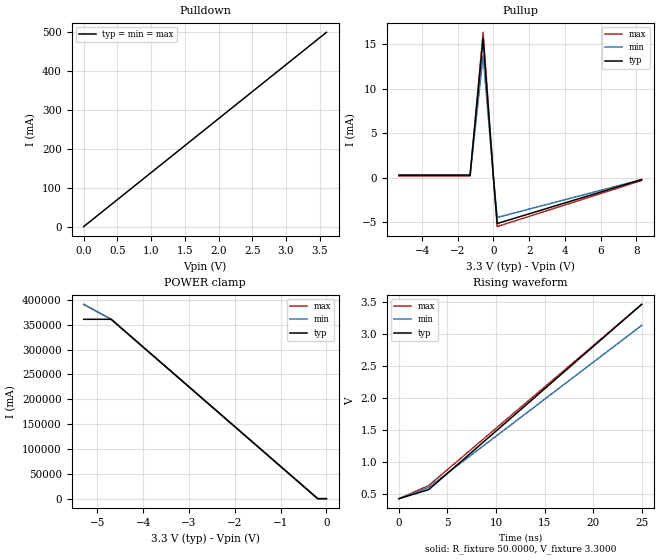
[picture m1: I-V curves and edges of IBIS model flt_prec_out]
[IBIS Ver]  2.1
[File Name] bug28.ibs
[File Rev]  1.0
[Date]   Fri Mar 27 11:24:04 1998
[Source]   IBIS_BUG
[Component]   comp
[Manufacturer]  fake
[Package]
| variable   typ   min   max
R_pkg   122.90m   NA   NA
L_pkg   10.33nH   NA   NA
C_pkg   0.82pF   NA   NA
[Pin] signal_name   model_name   R_pin L_pin  C_pin
1   sig   flt_prec_out   122.90m 10.33nH  0.82pF
2   VCC   POWER   122.90m 10.33nH  0.82pF
3   GND   GND   122.90m 10.33nH  0.82pF
| Models and submodels in the file (1): flt_prec_out (Output)
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[Model]   flt_prec_out
Model_type   Output
Vmeas = 1.5000
Cref = 5.00e-11
Rref = 50
Vref = 3.3
C_comp   0.5900pF   NA   NA
[Temperature Range]   50.00   50.0   50.0
[Voltage Range]   3.3000   3.0000   3.6000
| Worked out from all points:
|   slope of the pulldown table from 0 to 0.495 V, typ, clamps not added: 7.2 ohm
|   slope of the pullup table from 0 to 0.495 V, typ, clamps not added: 100 ohm
|   rising waveform, R_fixture 50.0000, V_fixture 3.3000: 20-80 % time 13.8ns typ, 14.1ns min, 14.1ns max; typ from 0.42 V to 3.47 V
[Pulldown]
| voltage   I(typ)   I(min)   I(max)
0V        0A         0A         0A
3.6V      500mA      500mA      500mA
[Pullup]
| voltage   I(typ)   I(min)   I(max)
-5.3V     300uA      300uA      200uA
-1.31V    300uA      300uA      200uA
-580mV    15.6mA     13.7mA     16.3mA
-10mV     255uA      223uA      271uA
0V        0A         0A         0A
210mV     -5.12mA    -4.44mA    -5.46mA
8.3V      -200uA     -200uA     -300uA
[Ramp]
dV/dt_r   1.0/.9n 1.0/.9n 1.0/.9n
dV/dt_f   .8/.6n .8/.6n .8/.6n
[GND_Clamp]
|Voltage   I(typ)   I(min)   I(max)
0V        0A         0A         0A
3.22V     0A         0A         0A
[POWER_Clamp]
|Voltage   I(typ)   I(min)   I(max)
-5.3V     361A       391A       391A
-4.7V     361A       361A       361A
-190mV    0A         0A         0A
0V        0A         0A         0A
[Rising Waveform]
R_fixture = 50.0000
V_fixture = 3.3000
|Time   Typ(v)   Min(v)   Max(v)
0s        420mV      420mV      420mV
3.08ns    563.2mV    598mV      627.1mV
24.98ns   3.47V      3.14V      3.47V
